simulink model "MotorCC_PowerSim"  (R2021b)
settings: Solver=ode45  StartTime=0.0  StopTime=0.6  RelTol=1e-3  EnableMultiTasking=on
InitFcn:
  | %% Parâmetros elétricos do motor
  | La = 0.0051881;
  | Ra = 4.2433;
  | B = 0.00014087;
  | J = 3.955e-5;
  | K = 0.084889;
undefined symbols (not defined in the file or in its folder): A, constant, N, Torque, Va
libraries: spsDCMachineLib x1, spsDiodeLib x1, spsIGBTLib x1, spsDCVoltageSourceLib x1, simulink x1, spspowerguiLib x1

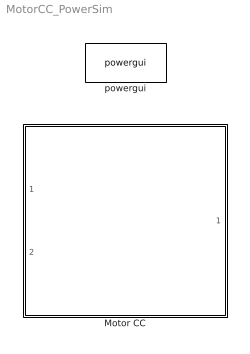
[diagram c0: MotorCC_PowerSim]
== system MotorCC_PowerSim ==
  Motor CC : Subsystem
  powergui : spspowerguiLib/powergui  Priority=1  SimulationMode=Continuous  SampleTime=50e-6  frequency=60  Iterations=50  frequencyindice=0  Pbase=100e6  ErrMax=1e-4  UnitsV=kV  UnitsW=MW  buscounter=0  FunctionMessages=off  echomessages=off  EnableUseOfTLC=off  CurrentSourceSwitches=off  DisableSnubberDevices=off  DisableRonSwitches=off  DisableVfSwitches=off  DisplayEquations=off  AutomaticDiscreteSolvers=off  SolverType=Tustin/Backward Euler (TBE)  Interpol=off  ExternalGateDelay=off  methode=off  Ts=100  x0status=blocks  SPID=on  SwTol=0  HookPort=off  NonlinearTolerance=1e-4  nMaxIteration=100  ContinueOnMaxIteration=off  RestoreLinks=warning  ResistiveCurrentMeasurement=off  Frange=[0:2:500]  Ylog=off  Xlog=on  ShowGrid=off  save=off  variable=ZData  structure=0  ZoomFFT=off  StartTime=0.0  cycles=1  DisplayStyle=1  fundamental=60  FreqAxis=off  MaxFrequency=1000  frequencyindicesteady=1  RmsSteady=1  display=off

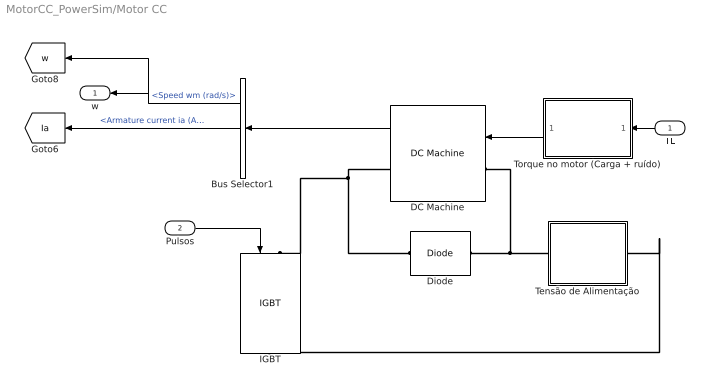
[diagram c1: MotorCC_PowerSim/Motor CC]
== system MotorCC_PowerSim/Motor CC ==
  TL : Inport
  Pulsos : Inport  Port=2
  Bus Selector1 : BusSelector  OutputSignals=Speed wm (rad/s),Armature current ia (A),Electrical torque Te (n m)
  DC Machine : spsDCMachineLib/DC Machine  PresetModel=No  MechanicalLoad=Torque TL  FieldType=Permanent magnet  ShowDetailedParameters=on  MeasurementBus=off  RLa=[Ra La]  RLf="[ 240  120]"  Laf=1.8  MachineConstant=Torque constant (N.m/A)  Ke=1.8  Kt=K  J=J  Bm=B  Tf=TC  w0=0  Ifinit=0  TsPowergui=0  TsBlock=-1
  Diode : spsDiodeLib/Diode  Ron=0.15  Lon=0  Vf=0.7  IC=0  UseSnubber=off  Rs=inf  Cs=inf  Measurements=off
  IGBT : spsIGBTLib/IGBT  Ron=0.01  Lon=0  Vf=0  Tf=1e-6  Tt=2e-6  IC=0  Rs=inf  Cs=inf  Measurements=off
  Tensão de Alimentação : Subsystem
  Torque no motor (Carga + ruído) : Subsystem
  w : Outport
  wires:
  TL/1 -> Torque no motor (Carga + ruído)/1(Carga)
  Pulsos/1 -> IGBT/1
  DC Machine/1 -> Bus Selector1/1
  Bus Selector1/1 -> [w], w/1  "<Speed wm (rad/s)>"
  Bus Selector1/2 -> [Ia]  "<Armature current ia (A)>"
  Torque no motor (Carga + ruído)/1(TL) -> DC Machine/1
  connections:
  Diode/LConn1 -- DC Machine/RConn1 -- IGBT/LConn1
  Diode/RConn1 -- DC Machine/LConn1 -- Tensão de Alimentação/LConn1
  IGBT/RConn1 -- Tensão de Alimentação/RConn1

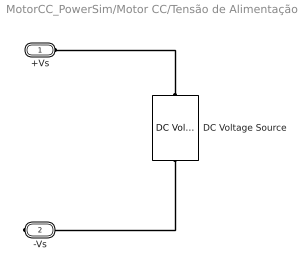
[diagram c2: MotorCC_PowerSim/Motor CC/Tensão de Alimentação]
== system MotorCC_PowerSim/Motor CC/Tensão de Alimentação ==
  DC Voltage Source : spsDCVoltageSourceLib/DC Voltage Source  Amplitude=Va  Measurements=None
  +Vs : PMIOPort  Side=Left
  -Vs : PMIOPort  Port=2  Side=Right
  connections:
  DC Voltage Source/RConn1 -- +Vs/RConn1
  DC Voltage Source/LConn1 -- -Vs/RConn1

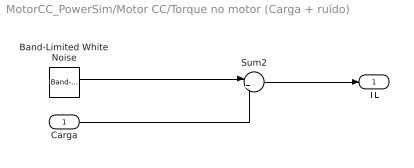
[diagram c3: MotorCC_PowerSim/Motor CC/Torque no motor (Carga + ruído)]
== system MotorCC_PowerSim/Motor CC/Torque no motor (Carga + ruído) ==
  Carga : Inport
  Band-Limited White Noise : simulink/Sources/Band-Limited White Noise  Cov=[0.00000001]  Ts=0.0000005  seed=[23341]
  Sum2 : Sum  Inputs=|++
  TL : Outport
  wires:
  Sum2/1 -> TL/1
  Carga/1 -> Sum2/2
  Band-Limited White Noise/1 -> Sum2/1
